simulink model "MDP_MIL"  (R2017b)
settings: Solver=FixedStepDiscrete  StartTime=0.0  StopTime=10.0  FixedStep=0.01  RelTol=1e-3  EnableMultiTasking=on
undefined symbols (not defined in the file): CcMDP_McuVoltFlt_V
libraries: AIWAYS_Powertrain_BMS_lib x7

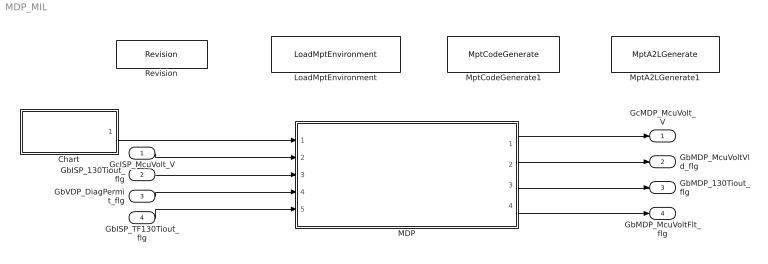
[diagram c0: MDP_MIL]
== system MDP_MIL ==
  GcISP_McuVolt_V : Inport
  GbISP_130Tiout_flg : Inport  Port=2
  GbVDP_DiagPermit_flg : Inport  Port=3
  GbISP_TF130Tiout_flg : Inport  Port=4
  Chart : Stateflow chart  TreatAsAtomicUnit=on
  LoadMptEnvironment : AIWAYS_Powertrain_BMS_lib/Config/LoadMptEnvironment  ProjectName=Comm  SuppierID=NewPlatformUAES
  MDP : Subsystem
  MptA2LGenerate1 : AIWAYS_Powertrain_BMS_lib/Config/MptA2LGenerate  SystemSampleTime=-1
  MptCodeGenerate1 : AIWAYS_Powertrain_BMS_lib/Config/MptCodeGenerate  SystemSampleTime=-1
  Revision : AIWAYS_Powertrain_BMS_lib/Config/Revision  curVersion='M101C101'  newVersion='M101C101'
  GcMDP_McuVolt_V : Outport
  GbMDP_McuVoltVld_flg : Outport  Port=2
  GbMDP_130Tiout_flg : Outport  Port=3
  GbMDP_McuVoltFlt_flg : Outport  Port=4
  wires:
  Chart/1(MDP_McuDataPrc_10ms()) -> MDP/1(MDP_McuDataPrc_10ms)
  GcISP_McuVolt_V/1 -> MDP/2(GcISP_McuVolt_V)
  GbISP_130Tiout_flg/1 -> MDP/3(GbISP_130Tiout_flg)
  MDP/1(GcMDP_McuVolt_V) -> GcMDP_McuVolt_V/1
  MDP/2(GbMDP_McuVoltVld_flg) -> GbMDP_McuVoltVld_flg/1
  GbVDP_DiagPermit_flg/1 -> MDP/4(GbVDP_DiagPermit_flg)
  MDP/3(GbMDP_130Tiout_flg) -> GbMDP_130Tiout_flg/1
  MDP/4(GbMDP_McuVoltFlt_flg) -> GbMDP_McuVoltFlt_flg/1
  GbISP_TF130Tiout_flg/1 -> MDP/5(GbISP_TF130Tiout_flg)

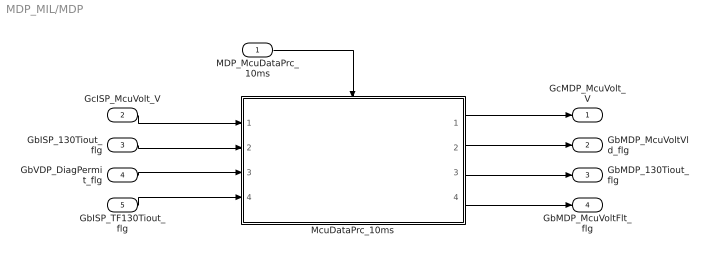
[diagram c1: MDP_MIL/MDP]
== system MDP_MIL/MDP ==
  MDP_McuDataPrc_10ms : Inport
  GcISP_McuVolt_V : Inport  Port=2
  GbISP_130Tiout_flg : Inport  Port=3
  GbVDP_DiagPermit_flg : Inport  Port=4
  GbISP_TF130Tiout_flg : Inport  Port=5
  McuDataPrc_10ms : Subsystem
  GcMDP_McuVolt_V : Outport
  GbMDP_McuVoltVld_flg : Outport  Port=2
  GbMDP_130Tiout_flg : Outport  Port=3
  GbMDP_McuVoltFlt_flg : Outport  Port=4
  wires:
  MDP_McuDataPrc_10ms/1 -> McuDataPrc_10ms/Trigger
  GcISP_McuVolt_V/1 -> McuDataPrc_10ms/1(GcISP_McuVolt_V)
  GbISP_130Tiout_flg/1 -> McuDataPrc_10ms/2(GbISP_130Tiout_flg)
  McuDataPrc_10ms/1(GcMDP_McuVolt_V) -> GcMDP_McuVolt_V/1
  McuDataPrc_10ms/2(GbMDP_McuVoltVld_flg) -> GbMDP_McuVoltVld_flg/1
  GbVDP_DiagPermit_flg/1 -> McuDataPrc_10ms/3(GbVDP_DiagPermit_flg)
  McuDataPrc_10ms/3(GbMDP_130Tiout_flg) -> GbMDP_130Tiout_flg/1
  McuDataPrc_10ms/4(GbMDP_McuVoltFlt_flg) -> GbMDP_McuVoltFlt_flg/1
  GbISP_TF130Tiout_flg/1 -> McuDataPrc_10ms/4(GbISP_TF130Tiout_flg)

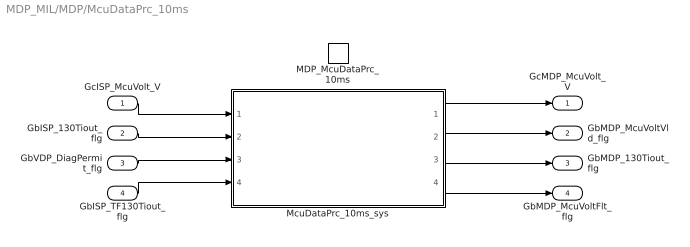
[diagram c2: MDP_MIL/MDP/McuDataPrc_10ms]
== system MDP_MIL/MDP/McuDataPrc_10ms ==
  GcISP_McuVolt_V : Inport
  GbISP_130Tiout_flg : Inport  Port=2
  GbVDP_DiagPermit_flg : Inport  Port=3
  GbISP_TF130Tiout_flg : Inport  Port=4
  MDP_McuDataPrc_10ms : TriggerPort  TriggerType=function-call  VariantControl=(inherit)
  McuDataPrc_10ms_sys : Subsystem
  GcMDP_McuVolt_V : Outport
  GbMDP_McuVoltVld_flg : Outport  Port=2
  GbMDP_130Tiout_flg : Outport  Port=3
  GbMDP_McuVoltFlt_flg : Outport  Port=4
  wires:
  GcISP_McuVolt_V/1 -> McuDataPrc_10ms_sys/1(GcISP_McuVolt_V)
  GbISP_130Tiout_flg/1 -> McuDataPrc_10ms_sys/2(GbISP_130Tiout_flg)
  McuDataPrc_10ms_sys/1(GcMDP_McuVolt_V) -> GcMDP_McuVolt_V/1
  McuDataPrc_10ms_sys/2(GbMDP_McuVoltVld_flg) -> GbMDP_McuVoltVld_flg/1
  GbVDP_DiagPermit_flg/1 -> McuDataPrc_10ms_sys/3(GbVDP_DiagPermit_flg)
  McuDataPrc_10ms_sys/3(GbMDP_130Tiout_flg) -> GbMDP_130Tiout_flg/1
  McuDataPrc_10ms_sys/4(GbMDP_McuVoltFlt_flg) -> GbMDP_McuVoltFlt_flg/1
  GbISP_TF130Tiout_flg/1 -> McuDataPrc_10ms_sys/4(GbISP_TF130Tiout_flg)

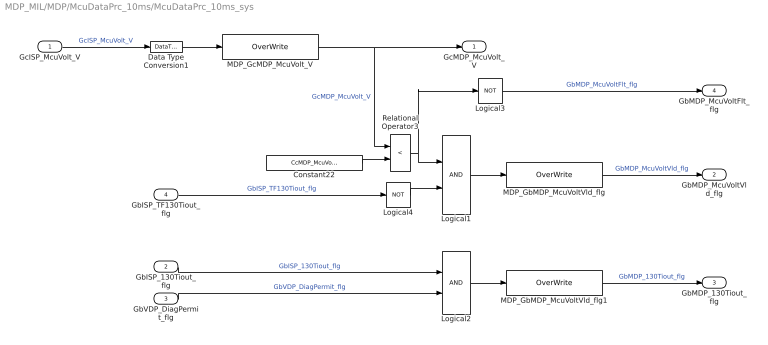
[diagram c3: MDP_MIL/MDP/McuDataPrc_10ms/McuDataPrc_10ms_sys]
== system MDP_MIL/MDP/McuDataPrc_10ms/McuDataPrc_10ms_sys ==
  GcISP_McuVolt_V : Inport
  GbISP_130Tiout_flg : Inport  Port=2
  GbVDP_DiagPermit_flg : Inport  Port=3
  GbISP_TF130Tiout_flg : Inport  Port=4
  Constant22 : Constant  Value=CcMDP_McuVoltFlt_V
  Data Type Conversion1 : DataTypeConversion
  Logical1 : Logic  OutDataTypeStr=boolean
  Logical2 : Logic  OutDataTypeStr=boolean
  Logical3 : Logic  Operator=NOT  OutDataTypeStr=boolean
  Logical4 : Logic  Operator=NOT  OutDataTypeStr=boolean
  MDP_GbMDP_McuVoltVld_flg : AIWAYS_Powertrain_BMS_lib/Signals/OverWrite  OverWrite_Value=CbMDP_McuVoltVldOvr_flg  OverWrite_flag=CbMDP_McuVoltVldOvrSwt_flg
  MDP_GbMDP_McuVoltVld_flg1 : AIWAYS_Powertrain_BMS_lib/Signals/OverWrite  OverWrite_Value=CbMDP_130TioutOvr_flg  OverWrite_flag=CbMDP_130TioutOvrSwt_flg
  MDP_GcMDP_McuVolt_V : AIWAYS_Powertrain_BMS_lib/Signals/OverWrite  OverWrite_Value=CcMDP_McuVoltOvr_V  OverWrite_flag=CbMDP_McuVoltOvrSwt_flg
  Relational Operator3 : RelationalOperator  Operator=<  OutDataTypeStr=boolean
  GcMDP_McuVolt_V : Outport
  GbMDP_McuVoltVld_flg : Outport  Port=2
  GbMDP_130Tiout_flg : Outport  Port=3
  GbMDP_McuVoltFlt_flg : Outport  Port=4
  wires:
  GbISP_130Tiout_flg/1 -> Logical2/1  "GbISP_130Tiout_flg"
  Logical1/1 -> MDP_GbMDP_McuVoltVld_flg/1
  GcISP_McuVolt_V/1 -> Data Type Conversion1/1  "GcISP_McuVolt_V"
  MDP_GbMDP_McuVoltVld_flg/1 -> GbMDP_McuVoltVld_flg/1  "GbMDP_McuVoltVld_flg"
  Data Type Conversion1/1 -> MDP_GcMDP_McuVolt_V/1
  MDP_GcMDP_McuVolt_V/1 -> Relational Operator3/1, GcMDP_McuVolt_V/1  "GcMDP_McuVolt_V"
  GbVDP_DiagPermit_flg/1 -> Logical2/2  "GbVDP_DiagPermit_flg"
  Logical2/1 -> MDP_GbMDP_McuVoltVld_flg1/1
  MDP_GbMDP_McuVoltVld_flg1/1 -> GbMDP_130Tiout_flg/1  "GbMDP_130Tiout_flg"
  Relational Operator3/1 -> Logical3/1, Logical1/1
  Logical4/1 -> Logical1/2
  Constant22/1 -> Relational Operator3/2
  Logical3/1 -> GbMDP_McuVoltFlt_flg/1  "GbMDP_McuVoltFlt_flg"
  GbISP_TF130Tiout_flg/1 -> Logical4/1  "GbISP_TF130Tiout_flg"

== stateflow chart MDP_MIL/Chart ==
  (default) -> (junction 1)
  (junction 1) -> (junction 3) : {MDP_McuDataPrc_10ms;}
  events: output FUNCTION_CALL_EVENT
